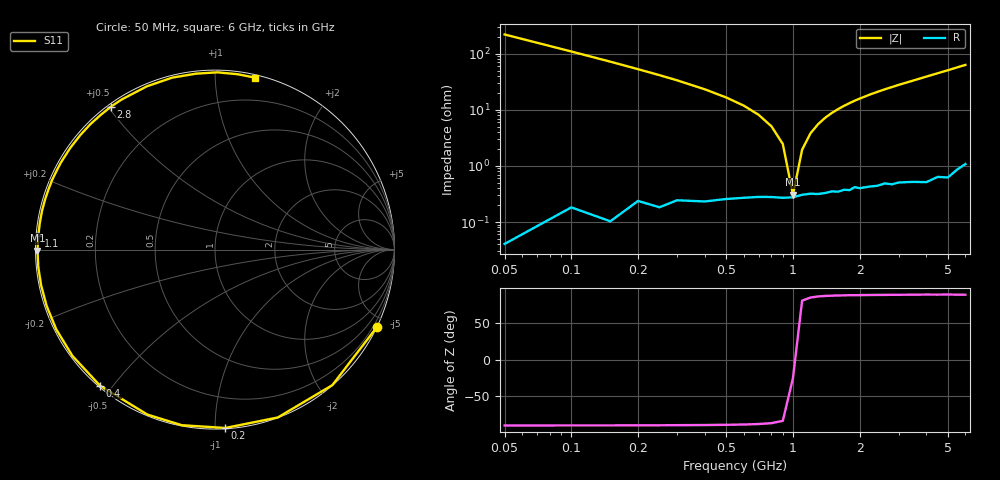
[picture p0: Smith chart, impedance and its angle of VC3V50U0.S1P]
! Infineon Technologies  Discrete & RF Semiconductors
! BBY 56-03
! Si Tuning Diode in SOD323
! VR = 3.5 V
! S-Parameters:  June  1999
# GHz  S  MA  R  50
!  f  S11
! GHz  MAG  ANG
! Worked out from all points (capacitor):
!   34 points, 50 MHz to 6 GHz, reference 50 ohm
!   read as one part to ground: C = 14.4 pF near 50 MHz
!   lowest |Z| = 305 mohm at 1 GHz (marker M1)
!   series resonance near 1.006 GHz, so ESL is about 1.7 nH
!   S11 on the Smith chart (normalised r, x): 50 MHz: 0.00, -4.40; 200 MHz: 0.00, -1.06; 400 MHz: 0.00, -0.46; 1.1 GHz: 0.01, +0.04; 2.8 GHz: 0.01, +0.51; 6 GHz: 0.02, +1.26
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0.05  0.9999 -25.6
0.1  0.9987 -49.1
0.15  0.9987 -69.5
0.2  0.9955 -86.7
0.25  0.9957 -100.7
0.3  0.9933 -112.3
0.4  0.9924 -130.2
0.5  0.9908 -143.3
0.6  0.9898 -153.3
0.7  0.9891 -161.5
0.8  0.989 -168.4
0.9  0.9893 -174.4
1  0.989 -179.7
1.1  0.9879 175.6
1.4  0.9871 163.5
1.6  0.9868 156.7
1.8  0.9862 150.5
2  0.9855 144.9
2.2  0.985 139.6
2.4  0.985 134.8
2.8  0.9852 126.0
3  0.9847 121.8
3.5  0.9857 112.6
4  0.9873 104.0
4.5  0.9859 96.2
5  0.9878 89.2
5.5  0.9852 82.6
6  0.9835 76.8
